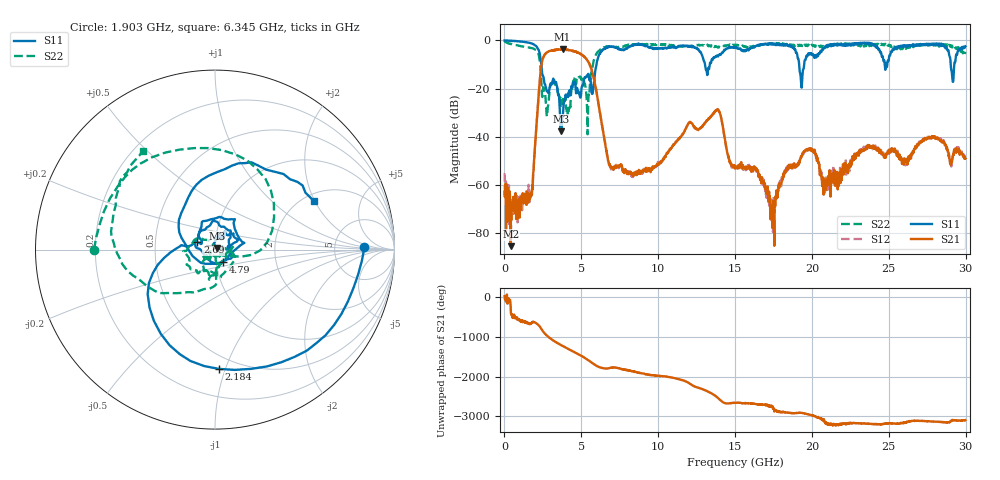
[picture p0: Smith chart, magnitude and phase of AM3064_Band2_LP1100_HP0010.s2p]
# Hz S DB R 50.0
!freq dBS11 angS11 dBS21 angS21 dBS12 angS12 dBS22 angS22
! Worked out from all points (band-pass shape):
!   1600 points, 10 MHz to 29.98 GHz, reference 50 ohm
!   highest |S21| = -3.66 dB at 3.777 GHz (marker M1); lowest = -85.3 dB at 403.6 MHz (marker M2)
!   |S21| within 3 dB of the highest: 2.552 GHz to 5.167 GHz (2.615 GHz wide, 67.7 % of centre)
!   lowest |S11| = -37.7 dB at 3.703 GHz (marker M3), VSWR 1.03, Z = 51 + j0.857 ohm
!   |S11| at or under -10 dB: 2.396 GHz to 5.983 GHz (3.587 GHz wide, 85.6 % of centre); 13.05 GHz to 13.35 GHz (303.9 MHz wide, 2.3 % of centre); 19.17 GHz to 19.49 GHz (324.5 MHz wide, 1.68 % of centre)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
!   |S22| runs from -38.9 to -0.3 dB; largest |S21 - S12| = 0.02
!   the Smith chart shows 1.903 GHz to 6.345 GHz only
!   S11 on the Smith chart (normalised r, x): 1.903 GHz: 11, +1; 2.184 GHz: 0.40, -0.95; 2.69 GHz: 0.82, +0.07; 4.79 GHz: 1.08, -0.15; 6.345 GHz: 2.25, +1.96
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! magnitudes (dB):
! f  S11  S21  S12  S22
! 10 MHz  0.0  -62.7  -55.0  -0.3
! 403.6 MHz  -0.1  -85.3  -70.9  -1.5
! 1.903 GHz  -1.6  -53.1  -52.0  -3.4
! 2.184 GHz  -3.5  -26.0  -26.0  -5.3
! 2.69 GHz  -19.5  -5.4  -5.4  -25.7
! 3.703 GHz  -37.7  -3.7  -3.8  -24.0
! 3.777 GHz  -31.6  -3.7  -3.8  -26.4
! 4.79 GHz  -21.8  -5.0  -5.0  -15.9
! 5.015 GHz  -19.8  -5.9  -5.8  -16.3
! 5.408 GHz  -14.3  -8.4  -8.4  -38.9
! 6.345 GHz  -4.3  -35.1  -34.9  -3.4
! 6.983 GHz  -2.6  -52.6  -53.0  -2.7
! 10 GHz  -3.4  -51.0  -51.1  -1.8
! 13.82 GHz  -6.3  -28.7  -28.7  -2.6
! 15 GHz  -2.8  -53.1  -52.2  -1.8
! 16.35 GHz  -2.4  -53.2  -52.8  -2.5
! 17.42 GHz  -1.7  -77.7  -66.4  -1.4
! 19.33 GHz  -19.6  -47.8  -48.0  -2.1
! 19.99 GHz  -5.4  -45.7  -45.6  -1.8
! 20.83 GHz  -3.2  -58.1  -63.3  -2.4
! 25 GHz  -8.1  -45.5  -45.9  -1.8
! 29.98 GHz  -2.5  -49.0  -48.4  -4.7
